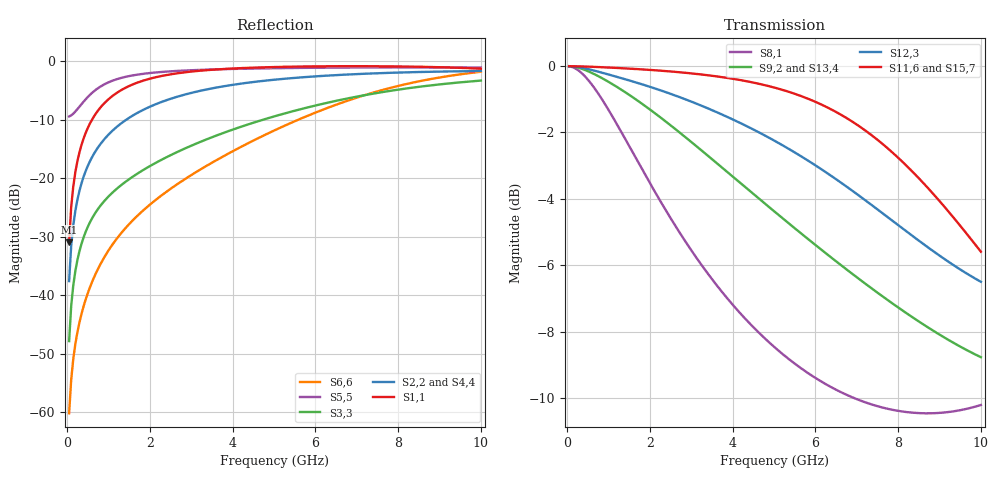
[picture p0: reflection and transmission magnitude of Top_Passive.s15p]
! Created Sat Dec 29 00:03:10 2018
! 15 Port Network Data from SP1.SP block
! freq  magS1_1  angS1_1  magS1_2  angS1_2  magS1_3  angS1_3  magS1_4  angS1_4
!  magS1_5  angS1_5  magS1_6  angS1_6  magS1_7  angS1_7  magS1_8  angS1_8
!  magS1_9  angS1_9  magS1_10  angS1_10  magS1_11  angS1_11  magS1_12  angS1_12
!  magS1_13  angS1_13  magS1_14  angS1_14  magS1_15  angS1_15
!  magS2_1  angS2_1
!  magS2_2  angS2_2  magS2_3  angS2_3  magS2_4  angS2_4  magS2_5  angS2_5
!  magS2_6  angS2_6  magS2_7  angS2_7  magS2_8  angS2_8  magS2_9  angS2_9
!  magS2_10  angS2_10  magS2_11  angS2_11  magS2_12  angS2_12  magS2_13  angS2_13
!  magS2_14  angS2_14  magS2_15  angS2_15
!  magS3_1  angS3_1  magS3_2  angS3_2
!  magS3_3  angS3_3  magS3_4  angS3_4  magS3_5  angS3_5  magS3_6  angS3_6
!  magS3_7  angS3_7  magS3_8  angS3_8  magS3_9  angS3_9  magS3_10  angS3_10
!  magS3_11  angS3_11  magS3_12  angS3_12  magS3_13  angS3_13  magS3_14  angS3_14
!  magS3_15  angS3_15
!  magS4_1  angS4_1  magS4_2  angS4_2  magS4_3  angS4_3
!  magS4_4  angS4_4  magS4_5  angS4_5  magS4_6  angS4_6  magS4_7  angS4_7
!  magS4_8  angS4_8  magS4_9  angS4_9  magS4_10  angS4_10  magS4_11  angS4_11
!  magS4_12  angS4_12  magS4_13  angS4_13  magS4_14  angS4_14  magS4_15  angS4_15
!  magS5_1  angS5_1  magS5_2  angS5_2  magS5_3  angS5_3  magS5_4  angS5_4
!  magS5_5  angS5_5  magS5_6  angS5_6  magS5_7  angS5_7  magS5_8  angS5_8
!  magS5_9  angS5_9  magS5_10  angS5_10  magS5_11  angS5_11  magS5_12  angS5_12
!  magS5_13  angS5_13  magS5_14  angS5_14  magS5_15  angS5_15
!  magS6_1  angS6_1
!  magS6_2  angS6_2  magS6_3  angS6_3  magS6_4  angS6_4  magS6_5  angS6_5
!  magS6_6  angS6_6  magS6_7  angS6_7  magS6_8  angS6_8  magS6_9  angS6_9
!  magS6_10  angS6_10  magS6_11  angS6_11  magS6_12  angS6_12  magS6_13  angS6_13
!  magS6_14  angS6_14  magS6_15  angS6_15
!  magS7_1  angS7_1  magS7_2  angS7_2
!  magS7_3  angS7_3  magS7_4  angS7_4  magS7_5  angS7_5  magS7_6  angS7_6
!  magS7_7  angS7_7  magS7_8  angS7_8  magS7_9  angS7_9  magS7_10  angS7_10
!  magS7_11  angS7_11  magS7_12  angS7_12  magS7_13  angS7_13  magS7_14  angS7_14
!  magS7_15  angS7_15
!  magS8_1  angS8_1  magS8_2  angS8_2  magS8_3  angS8_3
!  magS8_4  angS8_4  magS8_5  angS8_5  magS8_6  angS8_6  magS8_7  angS8_7
!  magS8_8  angS8_8  magS8_9  angS8_9  magS8_10  angS8_10  magS8_11  angS8_11
!  magS8_12  angS8_12  magS8_13  angS8_13  magS8_14  angS8_14  magS8_15  angS8_15
!  magS9_1  angS9_1  magS9_2  angS9_2  magS9_3  angS9_3  magS9_4  angS9_4
!  magS9_5  angS9_5  magS9_6  angS9_6  magS9_7  angS9_7  magS9_8  angS9_8
!  magS9_9  angS9_9  magS9_10  angS9_10  magS9_11  angS9_11  magS9_12  angS9_12
!  magS9_13  angS9_13  magS9_14  angS9_14  magS9_15  angS9_15
!  magS10_1  angS10_1
!  magS10_2  angS10_2  magS10_3  angS10_3  magS10_4  angS10_4  magS10_5  angS10_5
!  magS10_6  angS10_6  magS10_7  angS10_7  magS10_8  angS10_8  magS10_9  angS10_9
!  magS10_10  angS10_10  magS10_11  angS10_11  magS10_12  angS10_12  magS10_13  angS10_13
!  magS10_14  angS10_14  magS10_15  angS10_15
!  magS11_1  angS11_1  magS11_2  angS11_2
!  magS11_3  angS11_3  magS11_4  angS11_4  magS11_5  angS11_5  magS11_6  angS11_6
!  magS11_7  angS11_7  magS11_8  angS11_8  magS11_9  angS11_9  magS11_10  angS11_10
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# ghz S ma R 50
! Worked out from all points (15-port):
!   200 points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, 50 MHz to 10 GHz, reference 50 ohm
!   strongest paths, dB at 50 MHz, 2.55 GHz, 5.05 GHz, 7.55 GHz, 10 GHz:
!     S11,6: 0.0, -0.2, -0.7, -2.3, -5.6
!     S15,7: 0.0, -0.2, -0.8, -2.6, -5.9
!     S12,3: 0.0, -0.9, -2.3, -4.4, -6.5
!     S9,2: 0.0, -1.8, -4.4, -6.9, -8.8
!     S13,4: 0.0, -1.8, -4.5, -6.9, -8.8
!     S8,1: 0.0, -4.7, -8.5, -10.3, -10.2
!   lowest |S11| = -31.0 dB at 50 MHz (marker M1), VSWR 1.06, Z = 49.8 - j2.82 ohm
!   |S11| at or under -10 dB: start of sweep to 606.3 MHz
